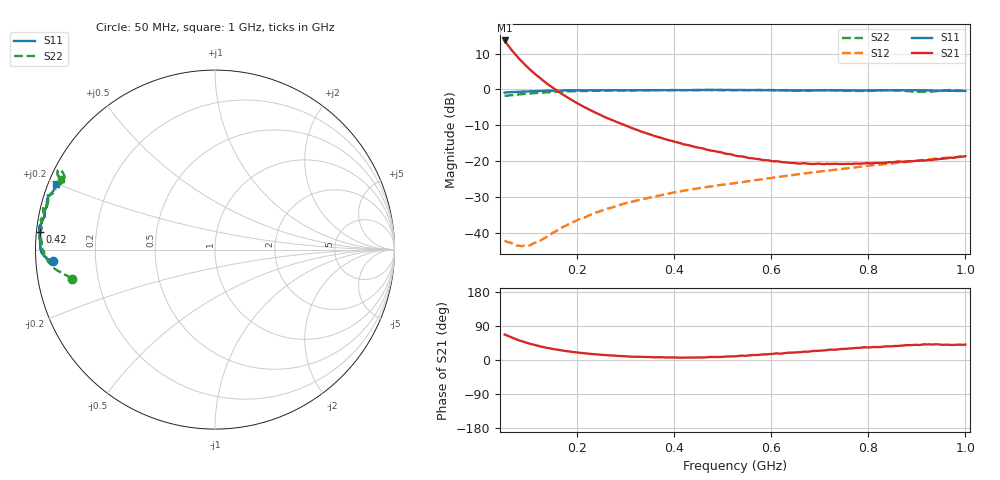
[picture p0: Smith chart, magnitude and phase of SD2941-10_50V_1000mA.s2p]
!Agilent Technologies,E8358A,US42080673,A.04.86
!Agilent E8358A: A.04.86
!Date: Friday, June 09, 2006 14:41:41
!Correction: S11(Full 2 Port SOLT,1,2) S21(Full 2 Port SOLT,1,2) S12(Full 2 Port SOLT,1,2) S22(Full 2 Port SOLT,1,2)
!S2P File: Measurements: S11, S21, S12, S22:
# Hz S  MA  R 50
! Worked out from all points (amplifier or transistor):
!   191 points, 50 MHz to 1 GHz, reference 50 ohm
!   highest |S21| = 13.7 dB at 50 MHz (marker M1)
!   |S21| within 3 dB of that: start of sweep to 66.53 MHz
!   unconditionally stable (mu >= 1): 770.9 MHz to 804.1 MHz; 881.5 MHz to 956.7 MHz; 990.4 MHz to end of sweep
!   at 205 MHz: K = 0.36, MSG = 16.0 dB, |S12| = -36.2 dB
!   at 525 MHz: K = 0.37, MSG = 3.8 dB, |S12| = -26.2 dB
!   at 1 GHz: K = 1.10, MAG = -1.9 dB, |S12| = -18.6 dB
!   S11 on the Smith chart (normalised r, x): 50 MHz: 0.05, -0.04; 420 MHz: 0.01, +0.05; 1 GHz: 0.02, +0.20
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5e7  0.9045 -175.8  4.841 67.3  0.007746 9.6  0.8141 -168.6
5.5e7  0.9124 -176.0  4.314 64.7  0.00742 10.4  0.8206 -168.9
6e7  0.9142 -176.2  3.896 61.8  0.007276 12.8  0.827 -169.3
6.5e7  0.9178 -176.2  3.526 59.0  0.007105 15.0  0.8335 -169.7
7.5e7  0.924 -176.5  2.933 54.1  0.006584 20.7  0.846 -170.4
8e7  0.9293 -176.7  2.685 51.8  0.006547 24.7  0.8522 -170.7
9e7  0.9354 -176.9  2.282 47.6  0.006564 33.5  0.8663 -171.3
1.05e8  0.9433 -177.5  1.825 42.0  0.006765 46.1  0.8818 -172.2
1.25e8  0.9534 -177.9  1.403 35.4  0.007826 59.3  0.9039 -173.5
1.5e8  0.9637 -178.8  1.045 28.9  0.01002 70.1  0.9218 -175.2
1.75e8  0.9685 -179.5  0.8091 23.9  0.01236 74.5  0.9376 -176.6
2.1e8  0.9728 179.6  0.5886 18.5  0.01616 78.3  0.9549 -178.5
2.7e8  0.9754 177.9  0.376 12.1  0.02226 79.3  0.9656 178.5
3.7e8  0.9806 175.8  0.2135 7.1  0.03301 78.2  0.977 174.1
4.2e8  0.9802 174.3  0.1705 6.4  0.03847 76.8  0.977 172.1
5.25e8  0.982 172.3  0.1193 9.6  0.04925 74.0  0.974 168.7
6.85e8  0.9722 168.3  0.09077 23.6  0.06945 69.9  0.9733 162.9
8.45e8  0.9738 163.8  0.09657 35.8  0.09187 65.1  0.9784 157.5
8.9e8  0.9758 162.5  0.09913 39.3  0.0992 63.6  0.9373 157.2
9.2e8  0.9674 161.6  0.1025 41.0  0.1051 63.1  0.9282 154.8
9.6e8  0.958 159.7  0.1087 40.4  0.1108 61.0  0.9751 152.8
1e9  0.9552 157.6  0.1171 40.5  0.1168 57.6  0.9425 155.3
